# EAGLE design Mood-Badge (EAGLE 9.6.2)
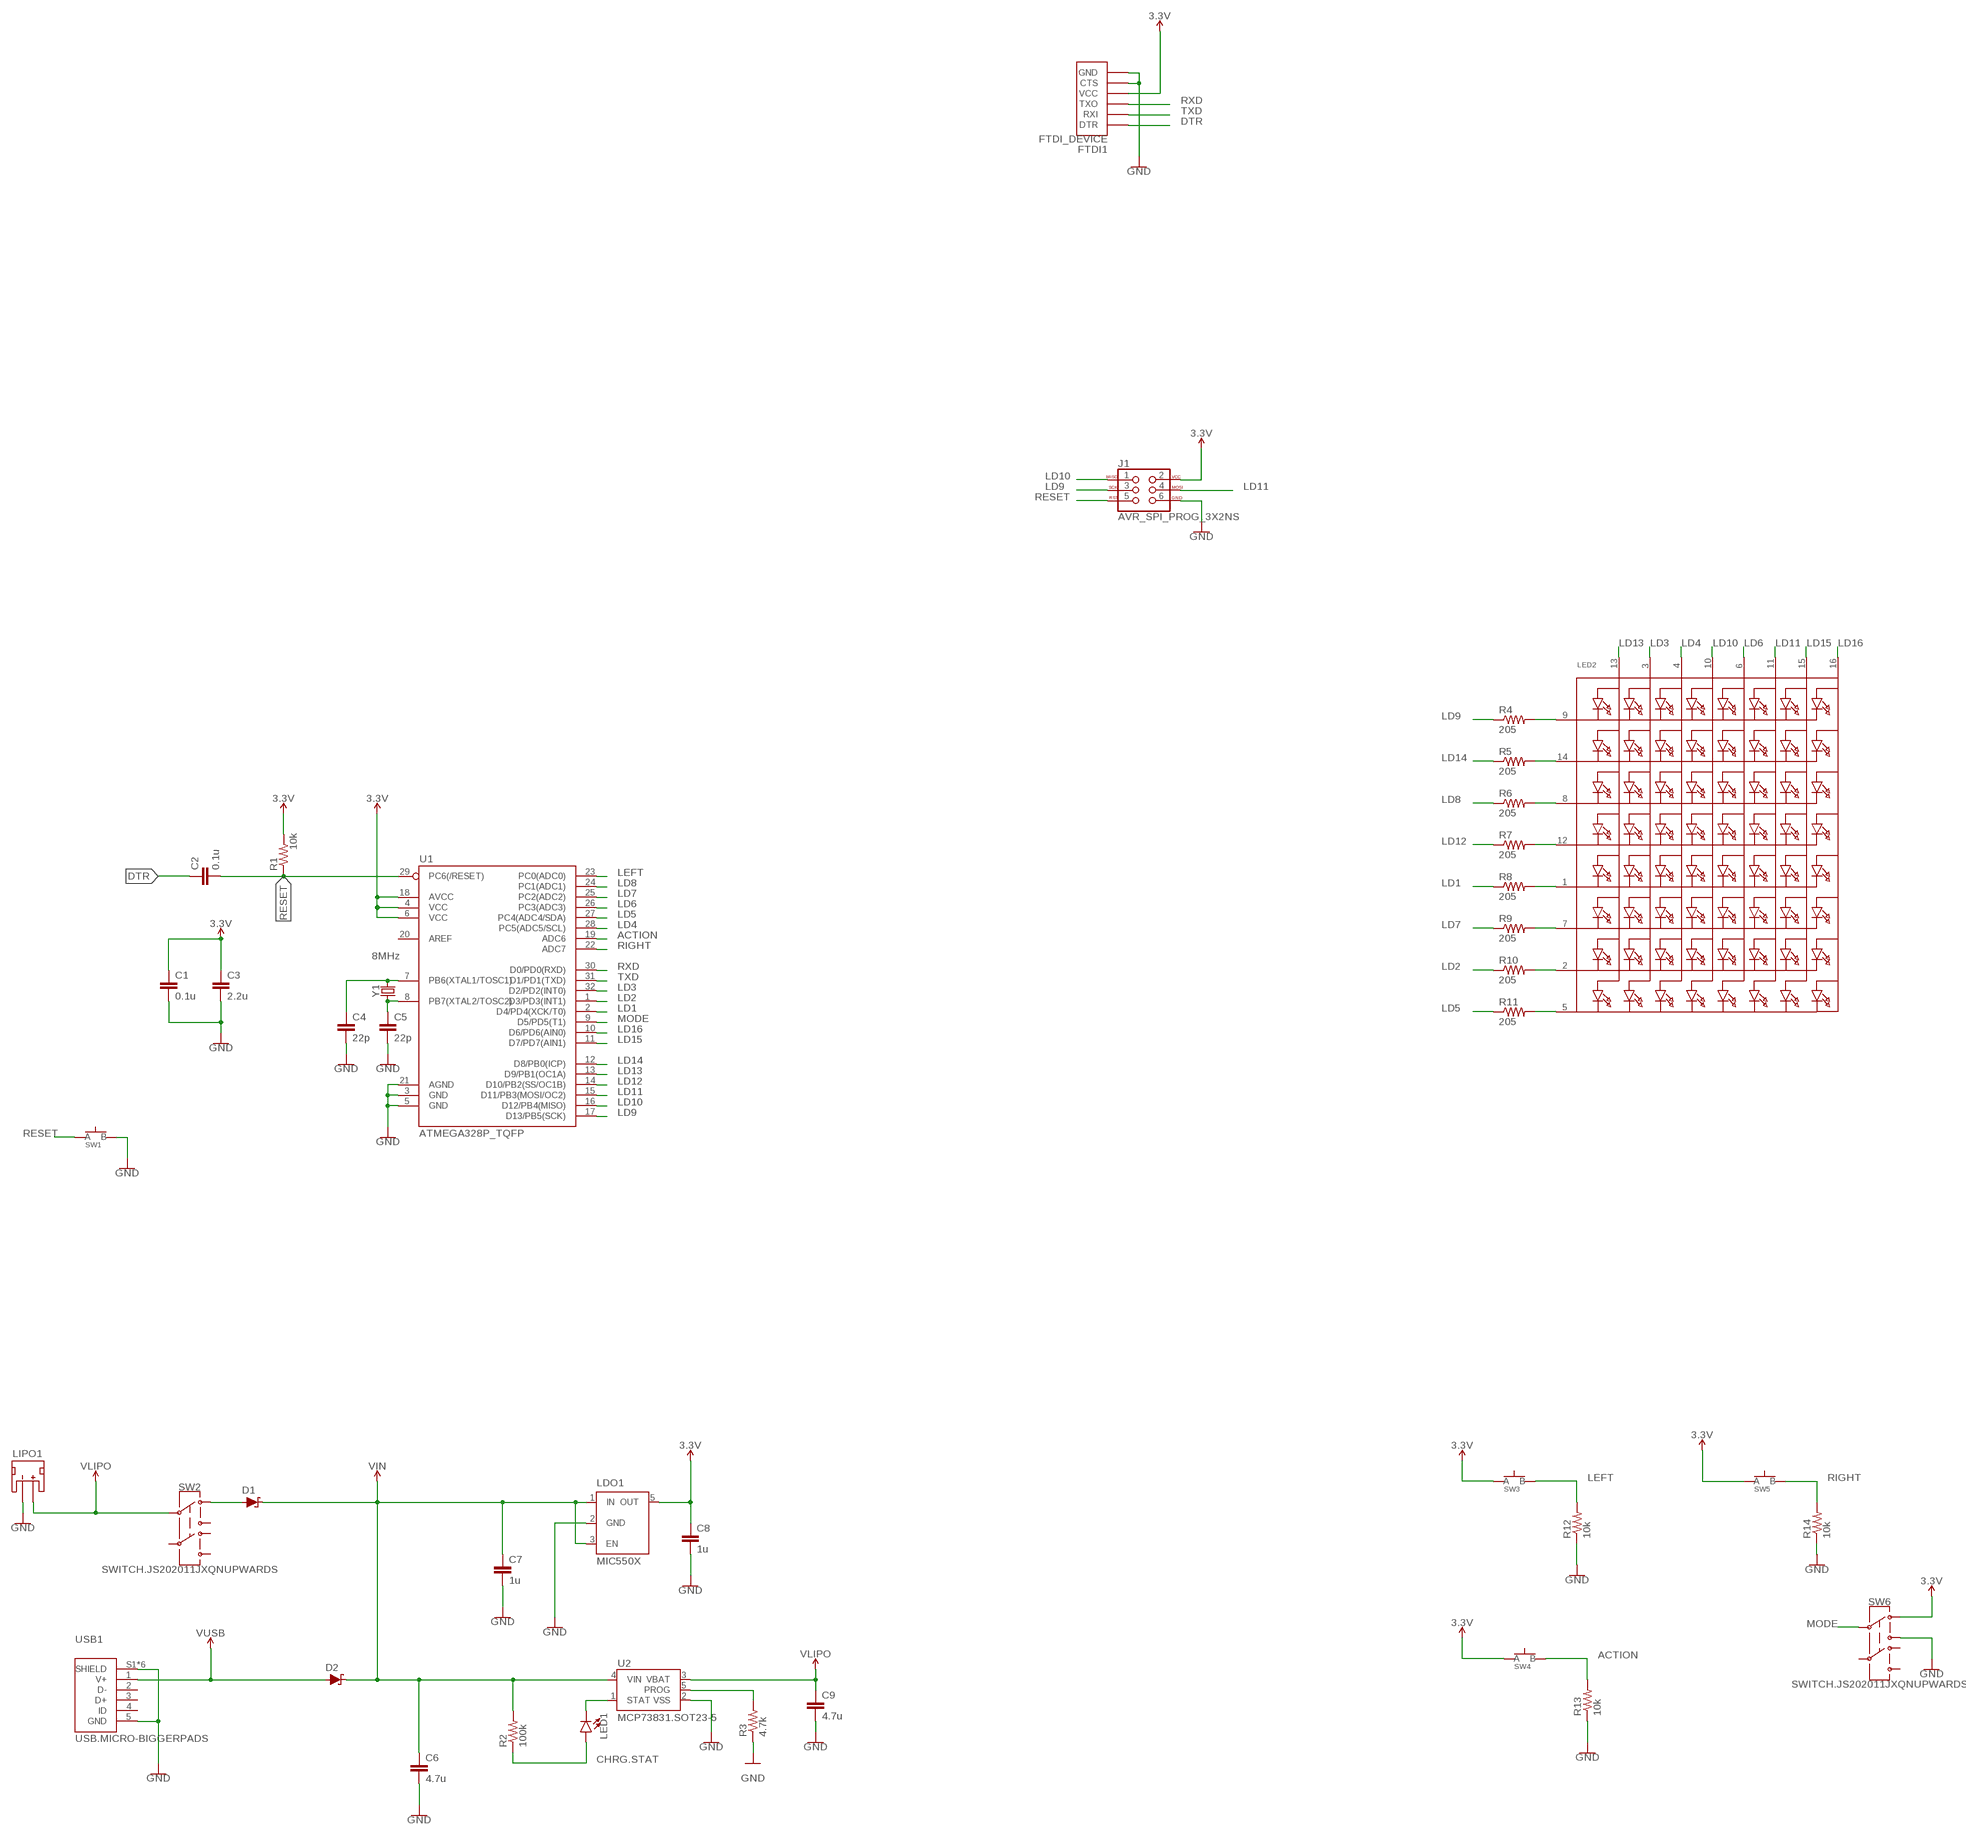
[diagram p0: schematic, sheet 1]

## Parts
C1  0.1u  CAPACITOR0603  [C0603]
C2  0.1u  CAPACITOR0603  [C0603]
C3  2.2u  CAPACITOR0603  [C0603]
C4  22p  CAPACITOR0603  [C0603]
C5  22p  CAPACITOR0603  [C0603]
C6  4.7u  CAPACITOR0603  [C0603]
C7  1u  CAPACITOR0603  [C0603]
C8  1u  CAPACITOR0603  [C0603]
C9  4.7u  CAPACITOR0603  [C0603]
D1  SCHOTTKY-USC  [USC]
D2  SCHOTTKY-USC  [USC]
FTDI1  FTDI_DEVICE  [FTDI_DEVICE]
J1  AVR_SPI_PROG_3X2NS  [2X3-NS]
LDO1  MIC550X  [SOT23-5]
LED1  LED0603  [LED-0603]
LED2  DOTMATRIX_8X8_ROWCATHODEM12A881UR  [DOTMATRIX_BL-M12A881UR]
LIPO1  JST_2MM_MALE  [JST-2-SMD]
R1  10k  RESISTOR0603  [R0603]
R2  100k  RESISTOR0603  [R0603]
R3  4.7k  RESISTOR0603  [R0603]
R4  205  RESISTOR0603  [R0603]
R5  205  RESISTOR0603  [R0603]
R6  205  RESISTOR0603  [R0603]
R7  205  RESISTOR0603  [R0603]
R8  205  RESISTOR0603  [R0603]
R9  205  RESISTOR0603  [R0603]
R10  205  RESISTOR0603  [R0603]
R11  205  RESISTOR0603  [R0603]
R12  10k  RESISTOR0603  [R0603]
R13  10k  RESISTOR0603  [R0603]
R14  10k  RESISTOR0603  [R0603]
SW1  SPST.KT11P4SM34LFS  [SPST.KT11P4SM34LFS]
SW2  SWITCH.JS202011JXQNUPWARDS  [SWITCH.00]
SW3  SPST.KT11P4SM34LFS  [SPST.KT11P4SM34LFS]
SW4  SPST.KT11P4SM34LFS  [SPST.KT11P4SM34LFS]
SW5  SPST.KT11P4SM34LFS  [SPST.KT11P4SM34LFS]
SW6  SWITCH.JS202011JXQNUPWARDS  [SWITCH.00]
U1  ATMEGA328P_TQFP  [TQFP32-08]
U2  MCP73831.SOT23-5  [SOT23-5]
USB1  USB.MICRO-BIGGERPADS  [USB-MICRO-01.BIGGERPADS]
Y1  8MHz  CRYSTAL-CA-310  [CA-301]

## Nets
3.3V: C1.1 C3.1 C8.1 FTDI1.VCC J1.2 LDO1.5(OUT) R1.2 SW3.1(A) SW3.2(A) SW4.1(A) SW4.2(A) SW5.1(A) SW5.2(A) SW6.1 U1.4(VCC) U1.6(VCC) U1.18(AVCC)
ACTION: R13.2 SW4.3(B) SW4.4(B) U1.19(ADC6)
CHRG.STAT: LED1.A R2.1
DTR: C2.1 FTDI1.DTR
GND: C1.2 C3.2 C4.2 C5.2 C6.2 C7.2 C8.2 C9.2 FTDI1.CTS FTDI1.GND J1.6 LDO1.2(GND) LIPO1.1(-) R3.1 R12.1 R13.1 R14.1 SW1.3(B) SW1.4(B) SW6.3 U1.3(GND) U1.5(GND) U1.21(AGND) U2.2(VSS) USB1.5(GND) USB1.S1(SHIELD) USB1.S2(SHIELD) USB1.S3(SHIELD) USB1.S4(SHIELD) USB1.S5(SHIELD) USB1.S6(SHIELD)
LD1: R8.1 U1.2(D4/PD4(XCK/T0))
LD2: R10.1 U1.1(D3/PD3(INT1))
LD3: LED2.3(A2) U1.32(D2/PD2(INT0))
LD4: LED2.4(A3) U1.28(PC5(ADC5/SCL))
LD5: R11.1 U1.27(PC4(ADC4/SDA))
LD6: LED2.6(A5) U1.26(PC3(ADC3))
LD7: R9.1 U1.25(PC2(ADC2))
LD8: R6.1 U1.24(PC1(ADC1))
LD9: J1.3 R4.1 U1.17(D13/PB5(SCK))
LD10: J1.1 LED2.10(A4) U1.16(D12/PB4(MISO))
LD11: J1.4 LED2.11(A6) U1.15(D11/PB3(MOSI/OC2))
LD12: R7.1 U1.14(D10/PB2(SS/OC1B))
LD13: LED2.13(A1) U1.13(D9/PB1(OC1A))
LD14: R5.1 U1.12(D8/PB0(ICP))
LD15: LED2.15(A7) U1.11(D7/PD7(AIN1))
LD16: LED2.16(A8) U1.10(D6/PD6(AIN0))
LEFT: R12.2 SW3.3(B) SW3.4(B) U1.23(PC0(ADC0))
MODE: SW6.2 U1.9(D5/PD5(T1))
N$3: C4.1 U1.7(PB6(XTAL1/TOSC1)) Y1.2
N$4: C5.1 U1.8(PB7(XTAL2/TOSC2)) Y1.1
N$6: LED1.C U2.1(STAT)
N$37: LED2.2(K7) R10.2
N$38: LED2.5(K8) R11.2
N$39: LED2.7(K6) R9.2
N$40: LED2.1(K5) R8.2
N$41: LED2.12(K4) R7.2
N$42: LED2.8(K3) R6.2
N$43: LED2.14(K2) R5.2
N$44: LED2.9(K1) R4.2
N$60: D1.+(A) SW2.1
N$64: R3.2 U2.5(PROG)
RESET: C2.2 J1.5 R1.1 SW1.1(A) SW1.2(A) U1.29(PC6(/RESET))
RIGHT: R14.2 SW5.3(B) SW5.4(B) U1.22(ADC7)
RXD: FTDI1.RXI(TXO) U1.30(D0/PD0(RXD))
TXD: FTDI1.TXO(RXI) U1.31(D1/PD1(TXD))
V_USB: D2.+(A) USB1.1(V+) ; supply symbol labelled VUSB
VIN: C6.1 C7.1 D1.-(C) D2.-(C) LDO1.1(IN) LDO1.3(EN) R2.2 U2.4(VIN)
VLIPO: C9.1 LIPO1.2(+) SW2.2 U2.3(VBAT)
Unconnected: LIPO1.NC1(PAD1) LIPO1.NC2(PAD2) SW2.3 SW2.5 SW2.6 SW2.7 SW6.5 SW6.6 SW6.7 U1.20(AREF) USB1.2(D-) USB1.3(D+) USB1.4(ID)

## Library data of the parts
C1-C9 = LinnesLab-Passives:CAPACITOR
D1 D2 = LinnesLab-DiscreteSemi:SCHOTTKY: Schottky diode
FTDI1 = LinnesLab-Connectors:FTDI_DEVICE
J1 = LinnesLab-Connectors:AVR_SPI_PROG_3X2: AVR ISP 6 Pin This is the reduced ISP connector for AVR programming. Common on Arduino. This footprint will take up less PCB space and can be used with a 10-pin to 6-pin adapter such as SKU: BOB-08508 **Special note about "TEST_POINT" package. The stop mask is on the top side, so if you want your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
LDO1 = LinnesLab-Power:MIC550X: MIC5504 Voltage Regulator Output Voltages: 1.0V to 3.3V Input Voltages: 2.5V to 5.5V Link to Datasheet http://ww1.microchip.com/downloads/en/DeviceDoc/MIC550X.pdf
LED1 = LinnesLab-LED:LED: LED (Generic)
LED2 = LinnesLab-Displays:DOTMATRIX_8X8_ROWCATHODE: 8x8 LED Segment Displays: Row = Cathode 0.7" Red 8X8 Matrix, 1.9mm Round LEDs - BL-M07C881UR 1.2" Red 8x8 Matrix, 3.0mm Round LEDs - BL-M12A881UR 1.2" Red 8x8 Matrix, 3.0mm Square LEDs - BL-M12A883
LIPO1 = LinnesLab-Connectors:JST_2MM_MALE: JST 2MM MALE RA CONNECTOR Two pin, compact surface mount connector. Commonly used as a battery input connection point. We really like the solid locking feeling and high current rating on these small connectors. We use these all the time as battery connectors. Mates to single-cell LiPo batteries.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; PROD_ID: CONN-11443; SF_ID: PRT-08612
R1-R14 = LinnesLab-Passives:RESISTOR
SW1 SW3-SW5 = LinnesLab-Switches:SPST.KT11P4SM34LFS: https://www.ckswitches.com/media/1468/kt.pdf
SW2 SW6 = LinnesLab-Switches:SWITCH.JS202011JXQN: Manufacturer's Part Numer: JS202011JAQN for right angle throw JS202011JCQN for top side throw
U1 = LinnesLab-Microcontrollers:ATMEGA328P_TQFP: Popular 328P in QFP Storefront component: ATmega328 - TQFP (COM-13448) Datasheet SparkFun Products SparkFun RedBoard - Programmed with Arduino (DEV-12757) Arduino Pro Mini 328 - 5V/16MHz (DEV-11113) Arduino Pro Mini 328 - 3.3V/8MHz (DEV-11114) SparkFun OpenLog (DEV-13712) SparkFun MicroView - OLED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; PROD_ID: IC-09069
U2 = LinnesLab-Power:MCP73831
USB1 = LinnesLab-Connectors:USB.MICRO: DigiKey PN: 609-4613-1-ND
Y1 = LinnesLab-Clocks:CRYSTAL-CA-310

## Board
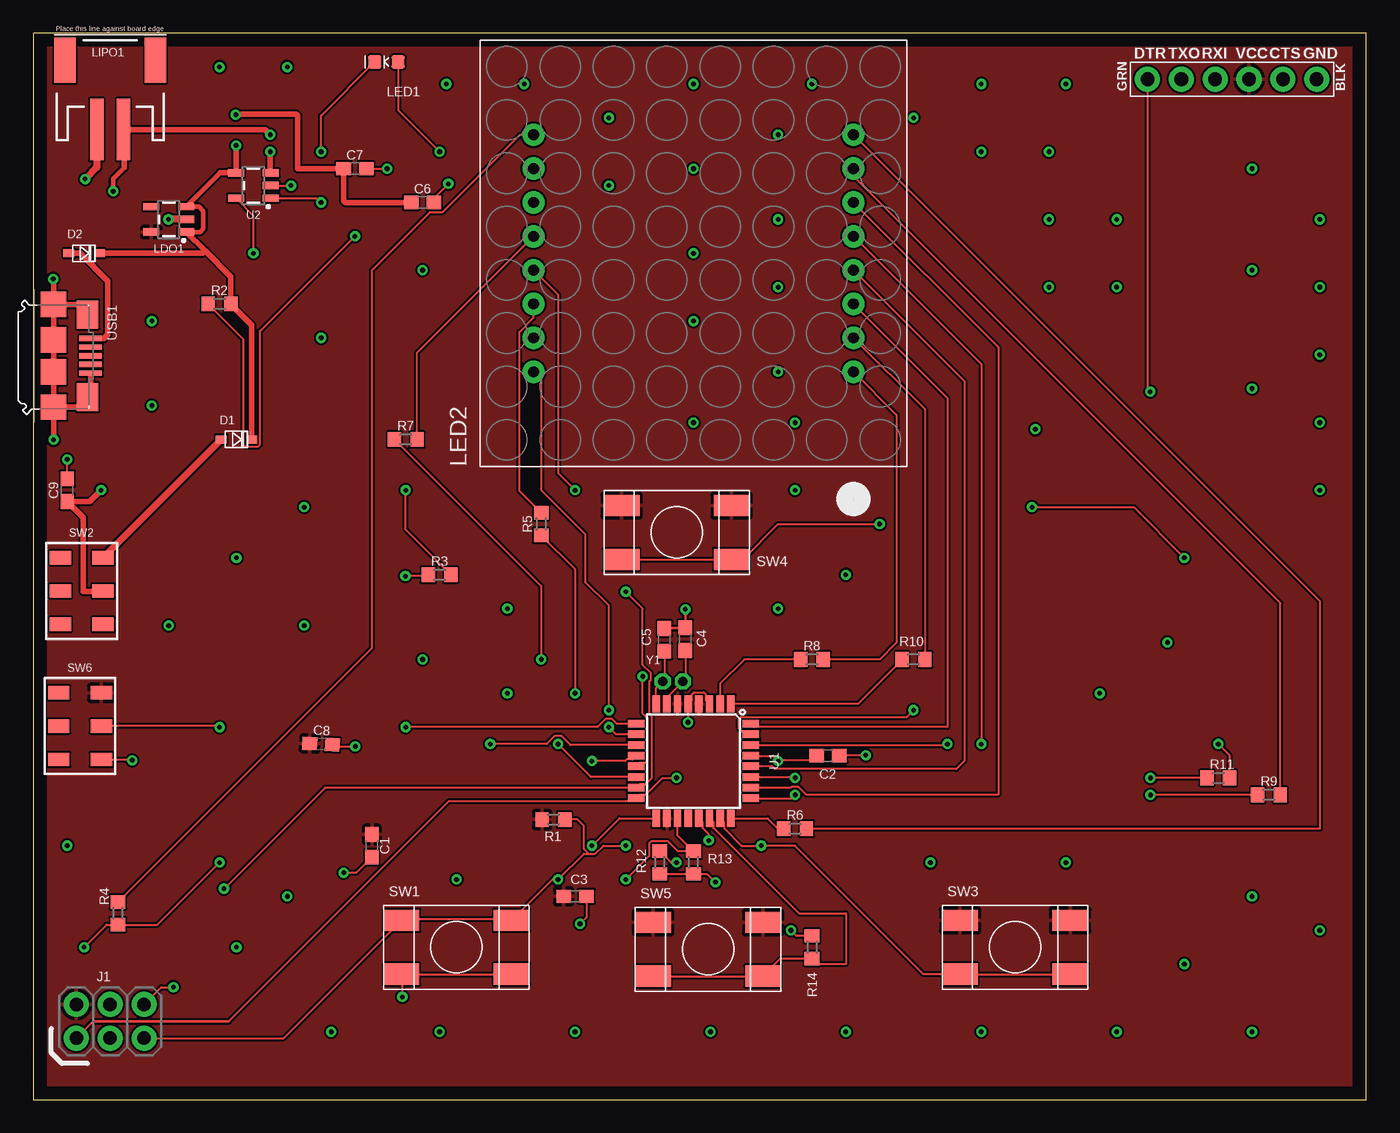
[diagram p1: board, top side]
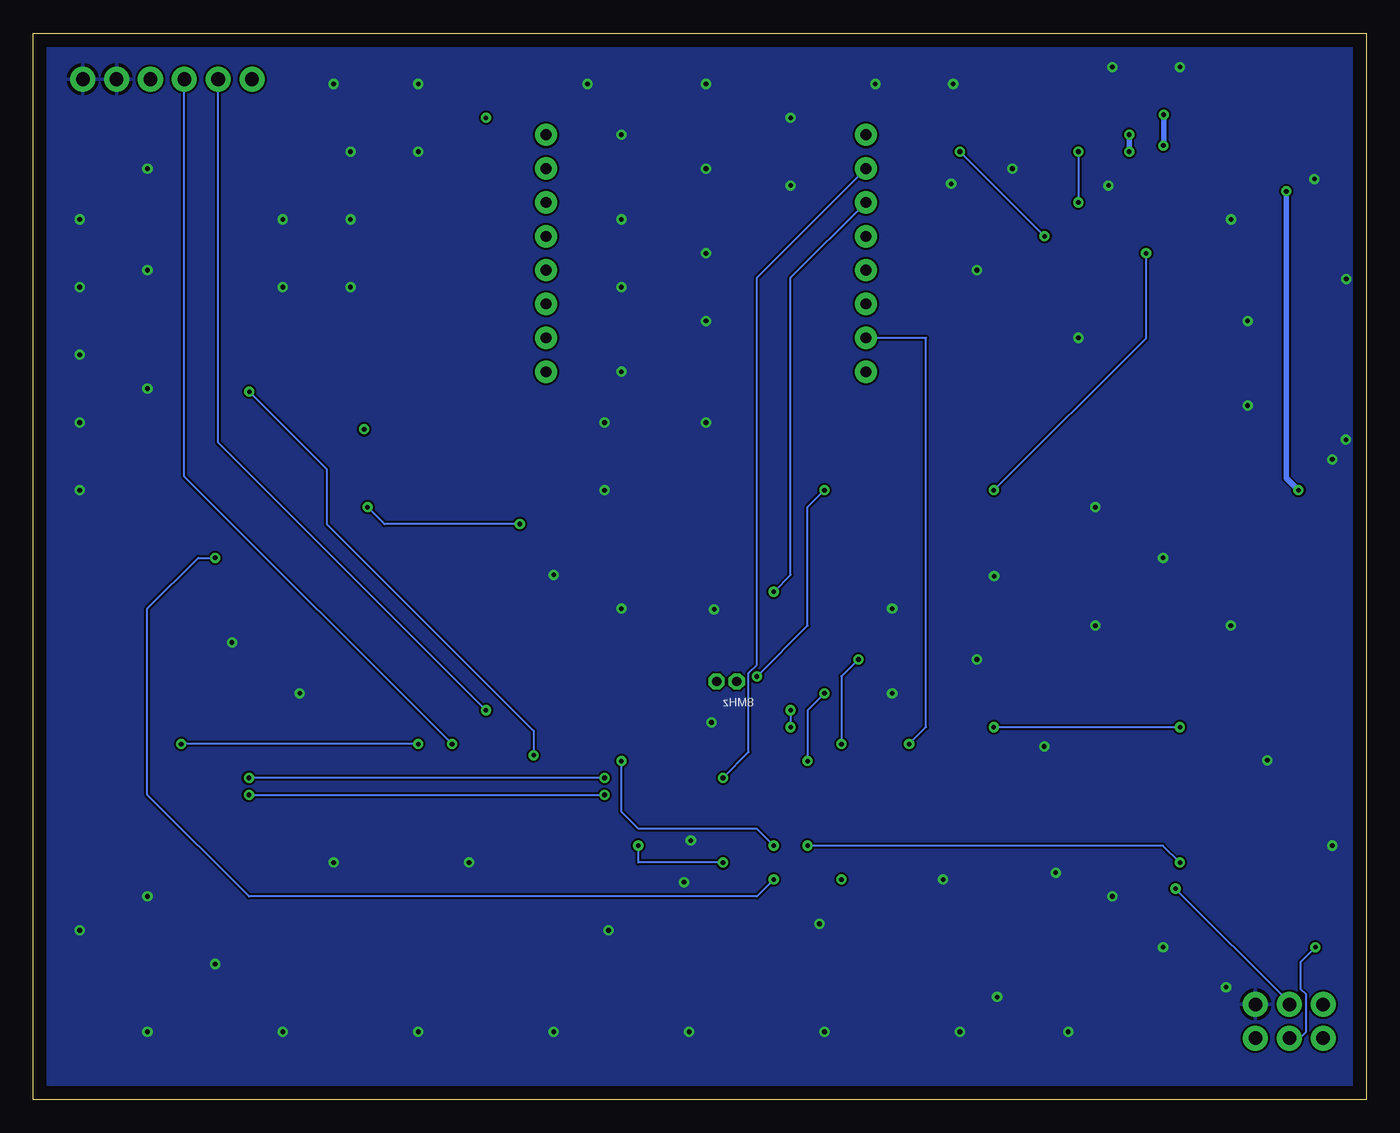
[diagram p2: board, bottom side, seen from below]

Size 100 x 80 mm. Coordinates in mm from the lower left corner, seen from the top.
Outline: 0,0 100,0 100,80 0,80 0,0
Copper layers (1*16): Top 0.035mm / dielectric 1.5mm / Bottom 0.035mm
Design rules "default": minimum track width 6mil, minimum drill 0.35mm, track to track 6mil, track to pad 6mil, pad to pad 6mil, via to via 6mil, smd to smd 6mil, copper to edge 40mil, drill to drill 6mil, minimum pad ring 10mil, minimum via ring 8mil, stop-mask expansion 4mil, vias tented up to drill 0mil, thermal gap 10mil

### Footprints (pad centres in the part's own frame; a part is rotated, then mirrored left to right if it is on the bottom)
C0603 = smd 1.1 x 1: 1 -0.85,0; 2 0.85,0
USC = smd 0.8 x 0.6: + -1.15,0; - 1.15,0
FTDI_DEVICE = drill 1.016 pad 1.88: CTS 3.81,0; DTR -6.35,0; GND 6.35,0; RXI -1.27,0; TXO -3.81,0; VCC 1.27,0
2X3-NS = drill 1.016 pad 1.88: 1 -2.54,-1.27; 2 -2.54,1.27; 3 0,-1.27; 4 0,1.27; 5 2.54,-1.27; 6 2.54,1.27
SOT23-5 = smd 0.55 x 1.2: 1 -0.95,-1.3; 2 0,-1.3; 3 0.95,-1.3; 4 0.95,1.3; 5 -0.95,1.3
LED-0603 = smd 1 x 1: A -0.877,0; C 0.877,0
DOTMATRIX_BL-M12A881UR = drill 0.8 pad 1.676: 1 -8.89,-12; 2 -6.35,-12; 3 -3.81,-12; 4 -1.27,-12; 5 1.27,-12; 6 3.81,-12; 7 6.35,-12; 8 8.89,-12; 9 8.89,12; 10 6.35,12; 11 3.81,12; 12 1.27,12; 13 -1.27,12; 14 -3.81,12; 15 -6.35,12; 16 -8.89,12
JST-2-SMD = smd 1 x 4.6: 1 -1,-3.7; 2 1,-3.7 | smd 1.6 x 3.4: NC1 -3.4,1.5; NC2 3.4,1.5
R0603 = smd 1 x 1.1: 1 -0.85,0; 2 0.85,0
SPST.KT11P4SM34LFS = smd 2.665 x 1.59: 1 -4.128,2.02; 2 4.128,2.02; 3 -4.128,-2.02; 4 4.128,-2.02
SWITCH.00 = smd 1 x 1.6: 1 -2.5,1.6; 2 0,1.6; 3 2.5,1.6; 5 -2.5,-1.6; 6 0,-1.6; 7 2.5,-1.6
TQFP32-08 = smd 1.27 x 0.559: 1 -4.293,2.8; 2 -4.293,2; 3 -4.293,1.2; 4 -4.293,0.4; 5 -4.293,-0.4; 6 -4.293,-1.2; 7 -4.293,-2; 8 -4.293,-2.8; 17 4.293,-2.8; 18 4.293,-2; 19 4.293,-1.2; 20 4.293,-0.4; 21 4.293,0.4; 22 4.293,1.2; 23 4.293,2; 24 4.293,2.8 | smd 0.559 x 1.27: 9 -2.8,-4.293; 10 -2,-4.293; 11 -1.2,-4.293; 12 -0.4,-4.293; 13 0.4,-4.293; 14 1.2,-4.293; 15 2,-4.293; 16 2.8,-4.293; 25 2.8,4.293; 26 2,4.293; 27 1.2,4.293; 28 0.4,4.293; 29 -0.4,4.293; 30 -1.2,4.293; 31 -2,4.293; 32 -2.8,4.293
USB-MICRO-01.BIGGERPADS = smd 0.4 x 1.7: 1 -1.3,1.505; 2 -0.65,1.505; 3 0,1.505; 4 0.65,1.505; 5 1.3,1.505 | smd 1.9 x 1.9: S1 -3.85,-1.27; S2 -1.2,-1.27; S3 1.2,-1.27; S4 3.85,-1.27 | smd 2.1 x 1.6: S5 -3.1,1.28; S6 3.1,1.28
CA-301 = drill 0.711 octagon: 1 0,0; 2 1.524,0

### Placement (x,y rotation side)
C1  25.4,19.05 270 top
C2  59.61,25.81 180 top
C3  40.64,15.24 0 top
C4  48.92,34.54 90 top
C5  47.35,34.49 90 top
C6  29.21,67.31 0 top
C7  24.13,69.85 0 top
C8  21.59,26.67 357 top
C9  2.54,45.72 90 top
D1  15.24,49.53 0 top
D2  3.81,63.5 0 top
FTDI1  89.94,76.56 0 top
J1  5.77,5.87 0 top
LDO1  10.16,66.04 90 top
LED1  26.49,77.85 180 top
LED2  49.53,63.5 90 top
LIPO1  5.77,76.48 0 top
R1  39.01,21.01 180 top
R2  13.97,59.69 0 top
R3  30.48,39.37 0 top
R4  6.35,13.97 90 top
R5  38.1,43.18 90 top
R6  57.15,20.32 0 top
R7  27.94,49.53 0 top
R8  58.42,33.02 0 top
R9  92.71,22.86 0 top
R10  66.04,33.02 0 top
R11  88.9,24.13 0 top
R12  46.99,17.78 90 top
R13  49.53,17.78 90 top
R14  58.42,11.43 270 top
SW1  31.75,11.43 0 top
SW2  3.63,38.15 270 top
SW3  73.66,11.43 0 top
SW4  48.26,42.55 0 top
SW5  50.62,11.28 0 top
SW6  3.51,28.02 270 top
U1  49.53,25.4 270 top
U2  16.51,68.58 90 top
USB1  2.79,55.8 270 top
Y1  47.22,31.37 0 top

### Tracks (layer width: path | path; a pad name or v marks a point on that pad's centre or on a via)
3.3V
  pour Top: 8.89,83.82 -3.81,83.82 -3.81,-5.08 -1.27,-5.08 104.14,-5.08 104.14,-3.81 104.14,82.55 104.14,83.82
ACTION  (via drill 0.35)
  Top 0.152: U1.19 48.33,19.83 R13.2 48.36,18.63 47.63,19.36 46.34,19.36 46.21,19.23 46.21,18.27 v44.45,16.51 | SW4.3 SW4.4 53.23,40.52 55.88,43.18 v63.5,43.18 | v74.93,44.45 82.55,44.45 v86.36,40.64
  Bottom 0.152: v44.45,16.51 45.72,15.24 83.82,15.24 91.44,22.86 91.44,36.83 87.63,40.64 v86.36,40.64 | v63.5,43.18 73.66,43.18 v74.93,44.45
CHRG.STAT  (via drill 0.35)
  Top 0.152: v24.13,64.77 17.02,57.66 17.02,49.13 16.89,49 15.89,49 15.76,49.13 15.76,57.05 R2.1 | LED1.A 27.37,74.23 v30.48,71.12
  Bottom 0.152: v24.13,64.77 v30.48,71.12
DTR  (via drill 0.35)
  Top 0.152: v83.8,53.11 83.59,53.31 FTDI1.DTR | v62.46,25.83 62.43,25.81 C2.1
  Bottom 0.152: v83.8,53.11 77.98,47.3 77.98,43.18 62.46,27.66 v62.46,25.83
GND  (via drill 0.35)
  Top 0.152: SW6.3 7.35,25.52 v7.42,25.45 | J1.6 9.6,8.43 v10.52,8.43 10.54,8.43 | C8.2 22.57,26.49 v24.16,26.49 | C1.2 24.22,17.02 v23.29,17.02 23.27,17.02 | SW1.4 SW1.3 27.69,9.35 v27.69,7.7 | C3.2 41.49,13.65 v41.02,13.18 | R12.1 R13.1 50.56,16.93 v51.18,16.31 | R14.1 57.27,12.28 v56.84,12.7 | R3.1 29.53,39.27 v27.91,39.27 27.89,39.27 | USB1.S6 4.04,52.67 3.32,51.95 | 1.52,61.54 v1.5,61.57 | C9.2 v2.54,48.03 2.54,48.06 | U2.2 v19.33,68.58 | C7.2 v26.54,69.85 26.57,69.85 | C6.2 30.06,67.63 v31.14,68.71 | U1.21 50.22,20.82 50.22,20.38 50.67,19.93 v50.67,19.43 50.67,19.38 | U1.3 50.44,29.98 50.44,30.42 50.3,30.56 49.56,30.56 49.42,30.42 49.42,29.98 U1.5 v49.13,28.3 v49.12,28.3
  Top 0.203: C5.2 47.4,35.39 C4.2 v48.92,36.78
  Top 0.406: USB1.S4 USB1.S3 USB1.S2 USB1.S1 | 3.32,51.95 USB1.S4 | USB1.S1 3.32,59.65 USB1.S5 | USB1.S1 1.52,61.54 | USB1.S4 v1.52,49.51 | USB1.5 4.3,52.93 4.04,52.67
  Top 0.508: LIPO1.1 4.77,69.94 v3.89,69.06 | LDO1.2 v10.13,66.04
  other vias: 2.54,19.05 30.48,5.08 40.64,5.08 50.8,5.08 60.96,5.08 71.12,5.08 81.28,5.08 91.44,5.08 96.52,12.7 91.44,15.24 86.36,10.16 77.47,17.78 67.31,17.78 80.01,30.48 85.09,34.29 96.52,45.72 96.52,50.8 96.52,55.88 96.52,60.96 96.52,66.04 91.44,69.85 91.44,62.23 91.44,53.34 81.28,60.96 81.28,66.04 76.2,60.96 76.2,66.04 76.2,71.12 77.47,76.2 71.12,76.2 71.12,71.12 19.05,77.47 13.97,77.47 21.59,57.15 29.21,62.23 8.89,58.42 8.89,52.07 20.32,44.45 15.24,40.64 10.16,35.56 20.32,35.56 57.15,50.8 55.88,54.61 49.53,50.8 49.53,58.42 49.53,63.5 55.88,60.96 55.88,66.04 55.88,72.39 58.42,76.2 49.53,76.2 49.53,69.85 43.18,68.58 43.18,73.66 36.83,76.2 35.56,36.83 29.21,33.02 55.88,36.83 60.96,39.37 57.15,45.72 31.75,16.51 19.05,15.24 15.24,11.43 35.56,30.48 30.99,76.2 22.35,5.08
  pour Bottom: 101.6,82.55 -1.27,82.55 -1.27,-2.54 101.6,-2.54
LD1
  Top 0.152: R8.1 53.34,33.02 51.53,31.21 U1.2
LD2
  Top 0.152: R10.1 61.86,29.69 U1.1
LD3
  Top 0.152: LED2.3 68.58,52.64 68.58,27.94 54.08,27.94 U1.32
LD4
  Top 0.152: LED2.4 69.85,53.91 69.85,25.4 69.24,24.79 55.63,24.79 55.42,25 U1.28
LD5  (via drill 0.35)
  Top 0.152: U1.27 57.08,24.2 v57.15,24.13 | R11.1 v83.82,24.13
  Bottom 0.152: v57.15,24.13 v83.82,24.13
LD6
  Top 0.152: LED2.6 72.39,56.45 72.39,22.86 58.01,22.86 57.4,23.47 56.9,23.47 56.83,23.4 U1.26
LD7  (via drill 0.35)
  Top 0.152: U1.25 56.89,22.6 v57.15,22.86 | R9.1 v83.82,22.86
  Bottom 0.152: v83.82,22.86 v57.15,22.86
LD8
  Top 0.152: R6.1 55.88,20.32 55.09,21.11 U1.24
LD9  (via drill 0.35)
  Top 0.152: v13.97,17.78 9.31,13.12 R4.1 5.5,13.12 v3.81,11.43 | v41.91,19.05 43.97,21.11 U1.17
  Bottom 0.152: J1.3 4.98,4.6 4.5,5.08 4.5,7.88 4.93,8.31 4.93,10.31 v3.81,11.43 | v13.97,17.78 15.24,19.05 v41.91,19.05
LD10  (via drill 0.35)
  Top 0.152: 14.66,5.87 31.18,22.4 45.03,22.4 U1.16 45.53,22.89 45.97,22.89 47.2,24.13 v48.26,24.13
  Top 0.203: J1.1 4.5,5.87 14.66,5.87
  Bottom 0.152: v48.26,24.13 46.33,26.06 46.33,32 45.72,32.61 45.72,61.66 LED2.10
LD11  (via drill 0.35)
  Top 0.152: v44.45,38.1 45.72,36.83 45.72,32.61 46.33,32 46.33,31.5 46.22,31.39 46.22,28.88 46.41,28.7 46.41,24.13 45.97,23.69 45.53,23.69 U1.15 21.88,23.4 v14.3,15.82
  Bottom 0.152: v44.45,38.1 43.18,39.37 43.18,61.66 LED2.11 | v14.3,15.82 5.77,7.29 J1.4
LD12  (via drill 0.35)
  Top 0.152: U1.14 41.84,24.2 v39.37,26.67 | R7.1 38.1,38.52 v38.1,33.02
  Bottom 0.152: v38.1,33.02 39.37,31.75 v39.37,26.67
LD13  (via drill 0.35)
  Top 0.152: LED2.13 39.37,60.39 39.37,46.99 v40.64,45.72 | U1.13 45.53,25.29 45.97,25.29 46.1,25.43 46.1,28.57 45.72,28.95 v45.72,31.75
  Bottom 0.152: v45.72,31.75 41.91,35.56 41.91,44.45 v40.64,45.72
LD14  (via drill 0.35)
  Top 0.152: R5.1 40.64,39.79 v40.64,30.48 | U1.12 44.95,25.51 44.51,25.51 44.4,25.4 v41.91,25.4
  Bottom 0.152: v40.64,30.48 41.91,29.21 v41.91,25.4
LD15  (via drill 0.35)
  Top 0.152: U1.11 40.3,26.6 39.62,27.28 39.12,27.28 38.51,26.67 v34.29,26.67
  Bottom 0.152: v34.29,26.67 33.02,27.94 33.02,57.15 LED2.15
LD16  (via drill 0.35)
  Top 0.152: LED2.16 38.1,54.04 38.1,45.72 41.4,42.42 41.4,38.85 43.18,37.07 v43.18,29.21 | U1.10 43.72,27.4 v43.18,27.94
  Bottom 0.152: v43.18,29.21 v43.18,27.94
LEFT  (via drill 0.35)
  Top 0.152: SW3.4 77.79,9.21 77.58,9.41 SW3.3 66.79,9.41 57.15,19.05 v54.61,19.05 53.15,19.05 51.82,20.38 51.82,20.82 U1.23 | R12.2 47.84,17.78 v48.26,17.78
  Bottom 0.152: v48.26,17.78 54.61,17.78 v54.61,19.05
MODE  (via drill 0.35)
  Top 0.152: SW6.2 13.89,28.02 v13.97,27.94 | U1.9 43.78,28.2 43.43,28.55 42.93,28.55 42.32,27.94 v27.94,27.94
  Bottom 0.152: v27.94,27.94 v13.97,27.94
N$1  (via drill 0.35)
  other vias: 66.04,73.66
N$2  (via drill 0.35)
  other vias: 75.18,50.29
N$3
  Top 0.152: U1.7 47.53,30.16 Y1.2 48.92,31.55 C4.1
N$4
  Top 0.152: U1.8 46.73,30.88 Y1.1 47.35,31.5 C5.1
N$6  (via drill 0.35)
  Top 0.152: LED1.C 21.59,73.83 v21.59,71.12 | U2.1 21.27,67.63 v21.59,67.31
  Bottom 0.152: v21.59,71.12 v21.59,67.31
N$37
  Top 0.152: LED2.2 66.89,51.79 R10.2
N$38  (via drill 0.35)
  Top 0.152: LED2.5 71.12,55.18 v71.12,26.67 | R11.2 89.75,25.82 v88.9,26.67
  Bottom 0.152: v71.12,26.67 v88.9,26.67
N$39
  Top 0.152: R9.2 93.56,37.25 61.53,69.28 LED2.7
N$40
  Top 0.152: LED2.1 64.77,51.37 64.77,34.29 63.5,33.02 R8.2
N$41
  Top 0.152: R7.2 28.79,56.03 LED2.12
N$42
  Top 0.152: LED2.8 96.52,37.4 96.52,20.32 R6.2
N$43
  Top 0.152: LED2.14 37.53,58.66 36.46,57.59 36.46,45.67 R5.2
N$44
  Top 0.152: R4.2 25.4,33.87 25.4,62.23 29.75,66.58 30.7,66.58 36.51,72.39 LED2.9
N$60
  Top 0.152: D1.+ 14.09,49.51
  Top 0.508: 14.09,49.51 SW2.1
N$64  (via drill 0.35)
  Top 0.152: R3.2 27.94,42.76 v27.94,45.72 | U2.5 16.51,66.33 v16.51,63.5
  Bottom 0.152: v27.94,45.72 16.51,57.15 v16.51,63.5
RESET  (via drill 0.35)
  Top 0.152: J1.5 18.77,4.6 SW1.1 27.72,13.55 35.98,13.55 | SW1.2 35.98,13.55 | 35.98,13.55 38.94,16.51 v39.37,16.51 41.3,18.44 41.66,18.44 | 41.66,18.44 41.3,18.8 41.3,20.55 40.84,21.01 R1.1 | 41.66,18.44 41.81,18.44 42.16,18.44 42.77,19.05 v44.45,19.05 | U1.29 55.48,25.8 55.83,25.45 | 55.83,25.45 v55.88,25.4 | C2.2 58.41,25.45 55.83,25.45
  Bottom 0.152: v44.45,19.05 45.72,20.32 54.61,20.32 55.88,21.59 v55.88,25.4
RIGHT
  Top 0.152: SW5.3 SW5.4 56.07,10.58 R14.2 58.84,10.16 60.96,10.16 60.96,13.97 57.43,13.97 51.02,20.38 51.02,20.82 U1.22
RXD  (via drill 0.35)
  Top 0.152: U1.30 68.51,26.6 v68.58,26.67
  Bottom 0.152: v68.58,26.67 88.67,46.76 FTDI1.RXI
TXD  (via drill 0.35)
  Top 0.152: v66.04,29.21 65.54,28.71 53.09,28.71 52.96,28.57 52.96,27.83 53.15,27.64 53.59,27.64 U1.31
  Bottom 0.152: v66.04,29.21 86.13,49.3 FTDI1.TXO
V_USB
  Top 0.406: USB1.1 5.29,57.1 5.59,57.4 5.59,61.42 3.5,63.5 D2.+
VIN  (via drill 0.35)
  Top 0.152: 12.7,63.5 12.88,63.67
  Top 0.356: LDO1.1 12.51,65.09 12.75,65.33 12.75,66.67 12.44,66.99 LDO1.3 14,69.53
  Top 0.406: D1.- 16.39,58.12 R2.2 14.82,61.73 12.88,63.67 LDO1.1 | 14,69.53 U2.4 v15.21,71.57 v15.21,71.58 | D2.- 12.7,63.5 | v15.19,73.89 15.21,73.91 19.74,73.91 19.84,73.81 19.84,69.85 C7.1 23.28,67.45 23.42,67.31 C6.1
  Bottom 0.406: v15.21,71.58 15.19,71.6 v15.19,73.89
VLIPO  (via drill 0.35)
  Top 0.152: U2.3 17.78,69.56 | 6.81,72.74 LIPO1.2 | 3.73,43.68 3.76,43.65 | 5.21,38.12 SW2.2
  Top 0.356: v5.99,68.15 5.99,69.09 6.81,69.9
  Top 0.406: LIPO1.2 17.39,72.78 v17.78,72.39 | 17.78,69.56 v17.78,71.12 | v5.08,45.72 4.23,44.87 C9.1 3.73,43.68 | 6.81,69.9 6.81,72.74 | 3.76,43.65 3.76,38.12 5.21,38.12
  Bottom 0.406: v17.78,72.39 v17.78,71.12 | v5.99,68.15 5.99,46.63 v5.08,45.72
